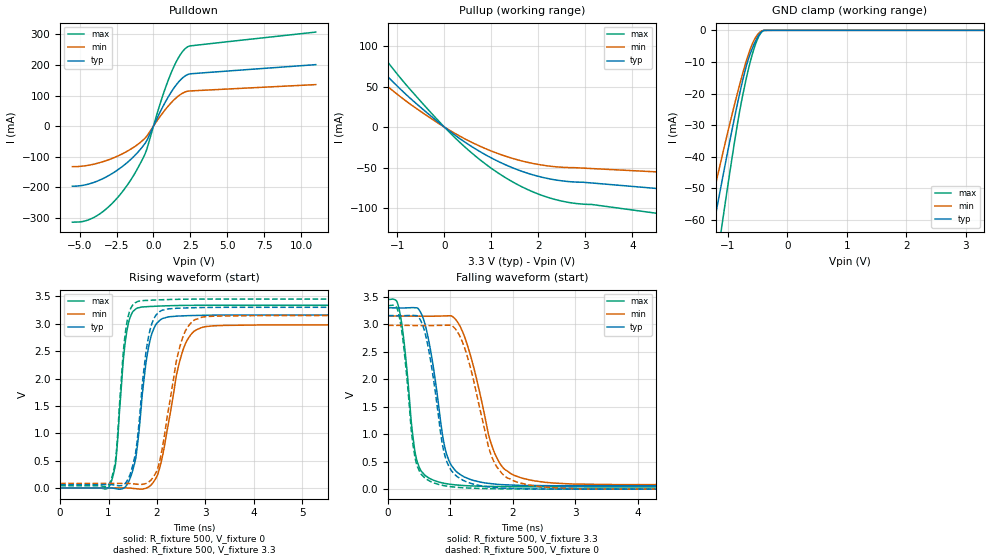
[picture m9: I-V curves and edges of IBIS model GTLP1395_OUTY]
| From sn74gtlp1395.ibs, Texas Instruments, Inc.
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[Model]   GTLP1395_OUTY
Model_type  3-state
Enable   Active-Low
Vref =   0
Rref =   500
Cref =   50p
Vmeas =   1.5
| variable   typ   min   max
C_comp   3.88pF   3.36pF   4.85pF
| C_pullup   4.40pF   3.63pF   5.41pF
| C_pulldown   6.11pF   3.61pF   8.49pF
| C_tri-state   3.88pF   3.36pF   4.85pF
[Temperature Range]   40   100   -40
| Ambient temperature   25   85   -40
[Voltage range]   3.3   3.15   3.45
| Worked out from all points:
|   slope of the pulldown table from 0 to 0.495 V, typ, clamps not added: 9.85 ohm
|   slope of the pullup table from 0 to 0.495 V, typ, clamps not added: 23.9 ohm
|   GND clamp passes 1 mA (typ) near -0.46 V on its own axis
|   rising waveform, R_fixture 500, V_fixture 0: 20-80 % time 241ps typ, 373ps min, 177ps max; typ from 0 V to 3.16 V
|   falling waveform, R_fixture 500, V_fixture 3.3: 20-80 % time 261ps typ, 400ps min, 179ps max; typ from 3.3 V to 0.061 V
|   rising waveform, R_fixture 500, V_fixture 3.3: 20-80 % time 234ps typ, 356ps min, 171ps max; typ from 0.061 V to 3.3 V
|   falling waveform, R_fixture 500, V_fixture 0: 20-80 % time 254ps typ, 383ps min, 176ps max; typ from 3.16 V to 0 V
[GND Clamp]
| GTLP1395_OUTY
|   Voltage   I(typ)   I(min)   I(max)
-5.5V     -550.2mA   -452.3mA   -722.5mA
-1.39V    -77.26mA   -64.32mA   -100.3mA
-1.335V   -71.56mA   -59.62mA   -92.84mA
-1.225V   -60.3mA    -50.36mA   -78.12mA
-1.125V   -50.27mA   -42.1mA    -64.99mA
-1.075V   -45.34mA   -38.05mA   -58.54mA
-845mV    -23.75mA   -20.27mA   -30.27mA
-700mV    -12.01mA   -10.31mA   -16.02mA
-540mV    -3.577mA   -2.435mA   -4.638mA
-470mV    -1.252mA   -725.2uA   -1.54mA
-410mV    -155uA     -70.07uA   -150.4uA
3.3V      299.8pA    27.28nA    -8.936nA
[Pulldown]
| GTLP1395_OUTY
|   Voltage   I(typ)   I(min)   I(max)
-5.5V     -196.7mA   -132.8mA   -314.5mA
-4.515V   -191.1mA   -129mA     -308.7mA
-3.555V   -174.7mA   -118.4mA   -284.4mA
-2.535V   -147mA     -100.3mA   -239.4mA
-1.56V    -110mA     -76mA      -177.8mA
-520mV    -52.85mA   -36.69mA   -84.85mA
510mV     51.71mA    35.63mA    81.99mA
1.215V    112.3mA    77.22mA    176.1mA
1.74V     146.4mA    100.3mA    227.6mA
2.22V     166.3mA    113mA      256.3mA
2.505V    171.2mA    115.1mA    262.7mA
11V       201.2mA    135.8mA    307.7mA
[Pullup]
| GTLP1395_OUTY
|   Voltage   I(typ)   I(min)   I(max)
-5.5V     323.6mA    255mA      420.5mA
-2.935V   166.7mA    134.2mA    214.7mA
-2.66V    149.8mA    120.6mA    192.8mA
-2.19V    120.9mA    97.36mA    155.8mA
-1.785V   96.39mA    77.52mA    124.2mA
-765mV    37.52mA    29.92mA    48.82mA
-45mV     2.077mA    1.636mA    2.736mA
480mV     -20.17mA   -15.77mA   -26.78mA
1.41V     -49.17mA   -37.84mA   -66.13mA
2.36V     -65.07mA   -48.83mA   -89.26mA
7.085V    -88.27mA   -62.85mA   -126.5mA
11V       -107.7mA   -74.59mA   -157.7mA
[Ramp]
| GTLP1395_OUTY
| variable   typ   min   max
dV/dt_r   1.91/2.52E-10   1.80/4.02E-10   2.01/1.90E-10
dV/dt_f   1.94/2.66E-10   1.84/4.14E-10   2.05/1.83E-10
R_load = 500
[Rising Waveform]
| GTLP1395_OUTY
R_fixture =   500
C_fixture =   0
L_fixture =   0
V_fixture =   0
V_fixture_min = 0
V_fixture_max = 0
|   Time   V(typ)   V(min)   V(max)
0s        -48.79nV   -110nV     114.4nV
1.03ns    1.733mV    98.56uV    57.36mV
1.145ns   -10.36mV   1.014mV    454.8mV
1.385ns   68.3mV     496.4uV    2.901V
1.56ns    537.5mV    -12.44mV   3.27V
1.69ns    1.658V     -19.57mV   3.307V
1.99ns    3.002V     199mV      3.321V
2.525ns   3.144V     2.488V     3.335V
2.985ns   3.155V     2.946V     3.338V
24.99ns   3.159V     2.979V     3.337V
[Falling Waveform]
| GTLP1395_OUTY
R_fixture =   500
C_fixture =   0
L_fixture =   0
V_fixture =   3.3
V_fixture_min = 3.15
V_fixture_max = 3.45
|   Time   V(typ)   V(min)   V(max)
0s        3.299V     3.15V      3.449V
195ps     3.296V     3.15V      3.175V
470ps     3.298V     3.148V     487.2mV
625ps     2.846V     3.146V     225.5mV
890ps     868.5mV    3.151V     108.6mV
1.03ns    407.3mV    3.142V     83.89mV
1.265ns   201mV      2.641V     62.35mV
1.775ns   85.79mV    499.4mV    47.09mV
2.52ns    63.47mV    124mV      42.15mV
24.99ns   60.96mV    84mV       40.15mV
[Rising Waveform]
| GTLP1395_OUTY
R_fixture =   500
C_fixture =   0
L_fixture =   0
V_fixture =   3.3
V_fixture_min = 3.15
V_fixture_max = 3.45
|   Time   V(typ)   V(min)   V(max)
0s        60.93mV    83.89mV    40.13mV
1.035ns   62.25mV    84mV       111.3mV
1.145ns   50.52mV    84.82mV    518.6mV
1.37ns    114.6mV    84.41mV    2.981V
1.635ns   1.247V     66.51mV    3.415V
1.785ns   2.556V     88.83mV    3.426V
1.96ns    3.132V     251.9mV    3.434V
2.5ns     3.286V     2.667V     3.448V
2.96ns    3.297V     3.126V     3.451V
24.99ns   3.3V       3.15V      3.45V
[Falling Waveform]
| GTLP1395_OUTY
R_fixture =   500
C_fixture =   0
L_fixture =   0
V_fixture =   0
V_fixture_min = 0
V_fixture_max = 0
|   Time   V(typ)   V(min)   V(max)
0s        3.158V     2.979V     3.337V
195ps     3.155V     2.979V     3.052V
465ps     3.155V     2.978V     425.9mV
615ps     2.732V     2.976V     182mV
875ps     786.2mV    2.981V     68.67mV
1.025ns   322mV      2.972V     42.48mV
1.25ns    136.7mV    2.488V     22.18mV
1.72ns    28.46mV    446.3mV    7.747mV
2.45ns    3.492mV    43.95mV    2.241mV
24.99ns   24.81uV    109.5uV    12.65uV
